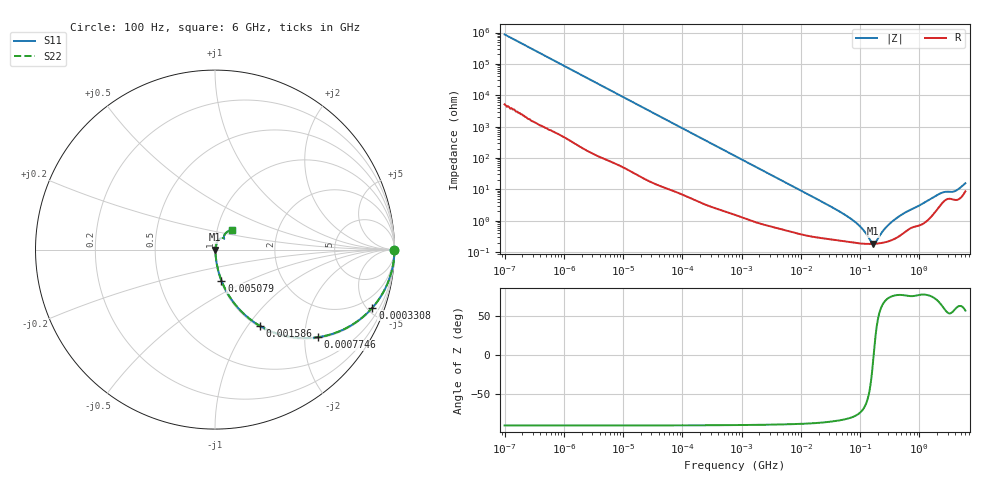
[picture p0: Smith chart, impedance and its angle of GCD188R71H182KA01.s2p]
!Murata Part Number: GCD188R71H182KA01
!These Parameters are Measured in Series Mode Connection
!Data Generated on Jan 08, 2026
!  o--ll--o
!Port1  Port2
!  o------o
!Operation Temp=25[degC], DC Bias Voltage=0[V]
!Freq. Start=100[Hz] Stop=6[GHz] 401[Steps]
# Hz S RI R 50
!Freq.(Hz) S11(Real) S11(Imag) S21(Real) S21(Imag) S12(Real) S12(Imag) S22(Real) S22(Imag)
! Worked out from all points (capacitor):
!   401 points, 100 Hz to 6 GHz, reference 50 ohm
!   read as one part in series: C = 1.83 nF near 109 Hz
!   lowest |Z| = 184 mohm at 166.9 MHz (marker M1)
!   series resonance near 169.7 MHz, so ESL is about 480 pH
!   S11 on the Smith chart (normalised r, x): 100 Hz: open; 330.8 kHz: 1.05, -5.40; 774.6 kHz: 1.03, -2.32; 1.586 MHz: 1.02, -1.14; 5.079 MHz: 1.01, -0.36; 6 GHz: 1.17, +0.26
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100  1 -0.000115  7e-07 0.000115  7e-07 0.000115  1 -0.000115
2008  1 -0.00229  1.64e-05 0.00229  1.64e-05 0.00229  1 -0.00229
40335  0.9977 -0.0454  0.00234 0.0454  0.00234 0.0454  0.9977 -0.0454
123542  0.98 -0.1359  0.02 0.1359  0.02 0.1359  0.98 -0.1359
330837  0.8771 -0.3235  0.1229 0.3235  0.1229 0.3235  0.8771 -0.3235
774597  0.5728 -0.4881  0.4272 0.4881  0.4272 0.4881  0.5728 -0.4881
1585629  0.2487 -0.4241  0.7513 0.4241  0.7513 0.4241  0.2487 -0.4241
2713602  0.1055 -0.2969  0.8945 0.2969  0.8945 0.2969  0.1055 -0.2969
5079039  0.036 -0.1724  0.964 0.1724  0.964 0.1724  0.036 -0.1724
1.555665e7  0.00655 -0.0585  0.9935 0.0585  0.9935 0.0585  0.00655 -0.0585
7.455971e7  0.00212 -0.0104  0.9979 0.0104  0.9979 0.0104  0.00212 -0.0104
1.066761e8  0.0019 -0.00549  0.9981 0.00549  0.9981 0.00549  0.0019 -0.00549
1.526266e8  0.00182 -0.00122  0.9982 0.00122  0.9982 0.00122  0.00182 -0.00122
1.669249e8  0.00183 -0.000186  0.9982 0.000186  0.9982 0.000186  0.00183 -0.000186
1.825626e8  0.00185 0.000847  0.9982 -0.000847  0.9982 -0.000847  0.00185 0.000847
2.497637e8  0.00203 0.00459  0.998 -0.00459  0.998 -0.00459  0.00203 0.00459
3.124326e8  0.00231 0.00752  0.9977 -0.00752  0.9977 -0.00752  0.00231 0.00752
5.346885e8  0.00419 0.0162  0.9958 -0.0162  0.9958 -0.0162  0.00419 0.0162
1.95892e9  0.0246 0.0582  0.9754 -0.0582  0.9754 -0.0582  0.0246 0.0582
2.562649e9  0.0432 0.0649  0.9568 -0.0649  0.9568 -0.0649  0.0432 0.0649
4.009986e9  0.049 0.0683  0.951 -0.0683  0.951 -0.0683  0.049 0.0683
6e9  0.0929 0.1095  0.9071 -0.1095  0.9071 -0.1095  0.0929 0.1095
